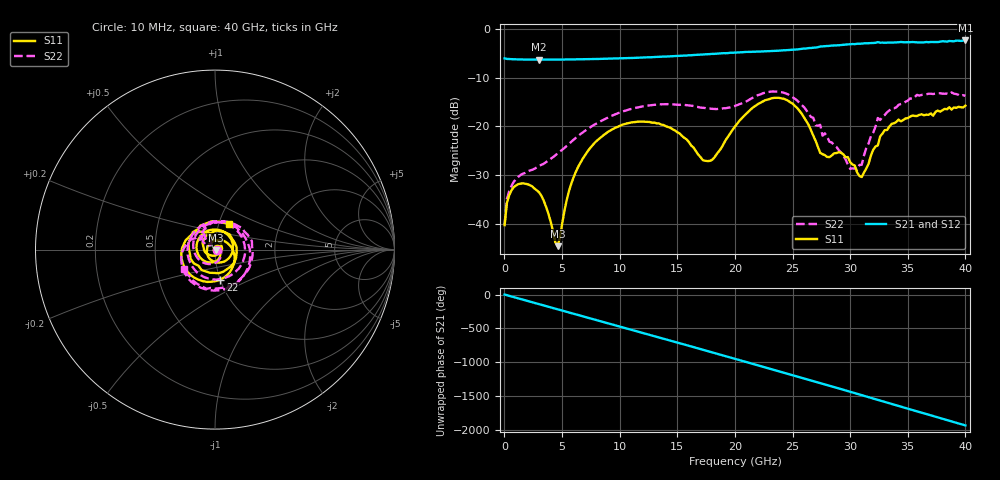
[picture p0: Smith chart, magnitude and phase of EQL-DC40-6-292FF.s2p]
!Agilent Technologies,N5230C,MY49001174,A.09.42.22
!Agilent N5230C: A.09.42.22
!Date: Wednesday, April 15, 2020 09:31:33
!Correction: S11(Full 2 Port(1,2))
!S21(Full 2 Port(1,2))
!S12(Full 2 Port(1,2))
!S22(Full 2 Port(1,2))
!S2P File: Measurements: S11, S21, S12, S22:
# Hz S  dB  R 50
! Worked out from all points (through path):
!   201 points, 10 MHz to 40 GHz, reference 50 ohm
!   highest |S21| = -2.37 dB at 40 GHz (marker M1); lowest = -6.3 dB at 3.009 GHz (marker M2)
!   group delay of S21, straight-line fit = 134 ps
!   lowest |S11| = -44.5 dB at 4.609 GHz (marker M3), VSWR 1.01, Z = 50.4 - j0.434 ohm
!   |S11| at or under -10 dB: start of sweep to end of sweep
!   |S22| runs from -40.0 to -12.8 dB; largest |S21 - S12| = 0.013
!   S11 on the Smith chart (normalised r, x): 10 MHz: 1.02, +0.00; 22 GHz: 1.00, -0.35; 40 GHz: 1.11, +0.33
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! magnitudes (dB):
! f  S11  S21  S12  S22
! 10 MHz  -40.2  -6.1  -6.1  -40.0
! 209.9 MHz  -35.6  -6.1  -6.1  -34.9
! 809.8 MHz  -32.4  -6.2  -6.2  -31.3
! 3.009 GHz  -33.5  -6.3  -6.3  -28.0
! 4.609 GHz  -44.5  -6.3  -6.3  -25.5
! 5.609 GHz  -33.1  -6.3  -6.3  -23.5
! 6.808 GHz  -26.5  -6.2  -6.2  -21.2
! 9.608 GHz  -20.3  -6.1  -6.1  -17.5
! 13.41 GHz  -19.4  -5.7  -5.7  -15.4
! 17.61 GHz  -27.1  -5.2  -5.2  -16.3
! 20 GHz  -20.0  -4.9  -4.9  -15.8
! 22 GHz  -15.4  -4.6  -4.6  -13.6
! 24.6 GHz  -14.7  -4.3  -4.3  -13.4
! 26.8 GHz  -21.8  -3.8  -3.8  -18.2
! 27.4 GHz  -25.4  -3.6  -3.6  -19.7
! 29.2 GHz  -25.4  -3.3  -3.3  -25.3
! 30.6 GHz  -29.4  -3.0  -3.1  -28.9
! 31 GHz  -30.4  -3.0  -3.0  -27.8
! 32.4 GHz  -23.9  -2.7  -2.7  -18.3
! 33.4 GHz  -20.0  -2.8  -2.8  -16.7
! 35.8 GHz  -17.9  -2.8  -2.8  -13.5
! 40 GHz  -15.7  -2.4  -2.3  -13.7
